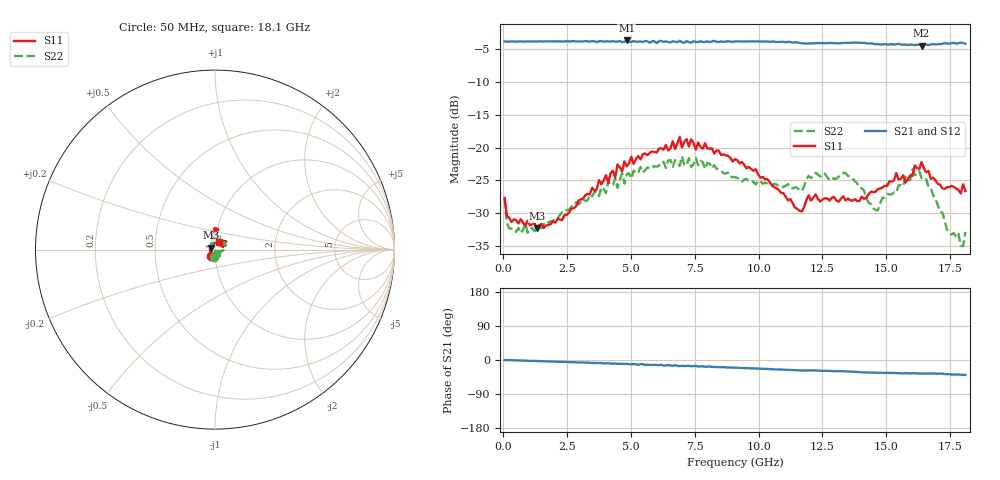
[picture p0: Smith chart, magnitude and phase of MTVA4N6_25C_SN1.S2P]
! Network Analyzer HP8720D.06.14 Serial No. US36140669
! 28 Jun 2005  13:34:56
! Frequency  S11  S21  S12  S22
# HZ  S  DB R 50
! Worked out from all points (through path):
!   201 points, 50 MHz to 18.1 GHz, reference 50 ohm
!   highest |S21| = -3.66 dB at 4.833 GHz (marker M1); lowest = -4.4 dB at 16.39 GHz (marker M2)
!   group delay of S21, straight-line fit = 6.19 ps
!   lowest |S11| = -32.3 dB at 1.313 GHz (marker M3), VSWR 1.05, Z = 47.8 + j1.01 ohm
!   |S11| at or under -10 dB: start of sweep to end of sweep
!   |S22| runs from -35.0 to -21.3 dB; largest |S21 - S12| = 0.02
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5e7  -27.64 -123.1  -3.81 -0.1  -3.81 0.3  -27.75 -96.5
1.4025e8  -30.38 -150.6  -3.84 -0.2  -3.84 -0.2  -31.53 -142.6
2.305e8  -30.70 -159.8  -3.84 -0.2  -3.83 -0.3  -32.27 -156.8
1.3135e9  -32.26 154.3  -3.82 -2.7  -3.81 -2.6  -32.12 152.4
3.1185e9  -27.79 100.0  -3.81 -6.6  -3.82 -6.8  -27.82 119.2
4.83325e9  -22.84 89.3  -3.66 -10.3  -3.77 -11.1  -24.04 92.6
6.09675e9  -20.15 83.6  -3.79 -13.5  -3.74 -13.5  -22.74 86.2
6.7285e9  -20.22 89.5  -3.87 -13.7  -4.00 -14.5  -21.88 79.1
6.909e9  -18.34 88.6  -3.69 -16.1  -3.81 -15.3  -22.79 76.7
6.99925e9  -19.98 87.5  -3.95 -15.2  -4.00 -16.5  -21.33 78.6
7.54075e9  -20.30 84.6  -3.87 -15.6  -3.75 -17.3  -21.58 81.6
9.075e9  -21.75 99.9  -3.81 -20.2  -3.80 -20.4  -24.47 62.3
1.1602e10  -29.61 105.2  -4.01 -27.4  -3.99 -27.7  -26.46 57.8
1.21435e10  -27.61 89.3  -4.10 -27.2  -4.07 -27.6  -24.35 58.4
1.3407e10  -28.05 55.9  -4.03 -29.9  -4.01 -30.2  -23.86 50.5
1.458025e10  -26.73 20.2  -4.22 -33.9  -4.16 -34.2  -29.50 53.4
1.512175e10  -25.15 25.3  -4.27 -34.1  -4.19 -34.2  -27.11 56.1
1.602425e10  -24.32 40.1  -4.28 -34.8  -4.41 -36.3  -23.30 36.0
1.638525e10  -22.19 36.2  -4.43 -35.7  -4.25 -35.7  -24.66 18.3
1.7378e10  -26.03 53.9  -4.12 -37.2  -3.98 -37.7  -32.51 -30.1
1.800975e10  -25.57 61.1  -4.06 -39.3  -4.06 -40.3  -35.01 -53.3
1.81e10  -26.60 59.1  -4.17 -39.3  -4.15 -40.2  -32.84 -66.2
